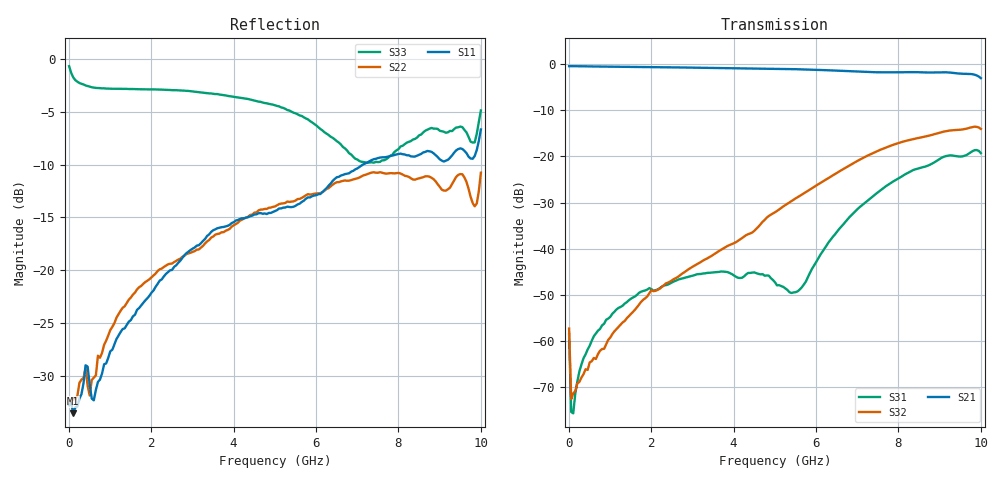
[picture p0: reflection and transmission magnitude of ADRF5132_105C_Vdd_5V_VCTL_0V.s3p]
! Device:  ADRF5132
! Description: Silicon SPDT Switch
! Frequency:  0.7 -  5 GHz
! Ports:
!	RFC	= Port 1
!	RF1	= Port 2
!  RF2  = Port 3
! Vdd:  5 Volt
! Control:  0/0 Volt
! Data:  Data was collected using a calibrated 4 port network analyzer and de-embedded using AtaiTec's In Situ De-Embedding.
! Note:  Analog Devices supplies this data as a sample of measured data
!  for this product.  Your particular data for this product may vary.
!  Data was taken at 105 degrees C.
!  Analog Devices reserves the right to change this data at anytime.
# GHZ S DB R 50.0
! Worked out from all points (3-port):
!   201 points, 10 MHz to 10 GHz, reference 50 ohm
!   strongest paths, dB at 10 MHz, 2.507 GHz, 5.005 GHz, 7.503 GHz, 10 GHz:
!     S21: -0.5, -0.7, -1.1, -1.8, -3.1
!     S32: -57.3, -46.8, -32.1, -18.8, -14.1
!     S31: -58.5, -47.3, -47.3, -27.8, -19.3
!   lowest |S11| = -33.5 dB at 109.9 MHz (marker M1), VSWR 1.04, Z = 52 - j0.735 ohm
!   |S11| at or under -10 dB: start of sweep to 7.143 GHz
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0.01  -32.74 16.0  -0.48 -0.1  -57.59 -59.4
      -0.48 -0.2  -32.76 21.9  -58.04 -54.3
      -58.46 -62.1  -57.26 -56.6  -0.70 -8.2
0.05995  -32.53 -9.4  -0.49 -1.0  -76.13 -31.5
         -0.49 -1.1  -32.37 -7.4  -72.39 -33.7
         -75.30 -45.1  -72.54 -33.3  -1.34 -42.6
0.1099  -33.52 -19.5  -0.50 -1.8  -75.44 34.4
        -0.49 -1.9  -32.22 -16.8  -71.88 -19.1
        -75.60 28.5  -71.29 -23.9  -1.76 -69.1
0.3097  -31.71 -32.9  -0.50 -5.1  -64.80 72.2
        -0.50 -5.1  -30.33 -31.9  -67.67 -43.6
        -65.02 70.6  -67.85 -48.1  -2.37 -128.1
0.75925  -30.33 -75.6  -0.56 -12.1  -57.38 80.6
         -0.56 -12.1  -28.26 -57.7  -62.01 -90.2
         -57.35 80.9  -62.07 -90.9  -2.78 -164.9
2.85715  -18.38 -149.7  -0.78 -44.3  -46.10 66.4
         -0.78 -44.3  -18.46 -113.4  -44.77 -166.0
         -46.17 66.1  -44.74 -165.9  -3.03 150.6
5.005  -14.40 155.9  -1.06 -77.0  -47.28 6.4
       -1.06 -77.1  -13.97 -136.7  -32.08 172.6
       -47.26 6.6  -32.08 172.8  -4.40 118.7
5.55445  -13.77 149.4  -1.15 -86.0  -49.15 -64.6
         -1.15 -86.0  -13.26 -142.5  -28.83 161.2
         -49.21 -63.8  -28.83 161.3  -5.25 110.5
9.6004  -8.70 70.7  -2.14 -151.6  -19.88 71.4
        -2.13 -151.7  -11.22 164.2  -14.08 37.8
        -19.88 71.5  -14.09 38.0  -6.73 98.9
10  -6.68 31.7  -3.08 -172.4  -19.31 25.4
    -3.07 -172.5  -10.78 117.5  -14.06 13.0
    -19.31 25.6  -14.07 13.2  -4.89 29.4
